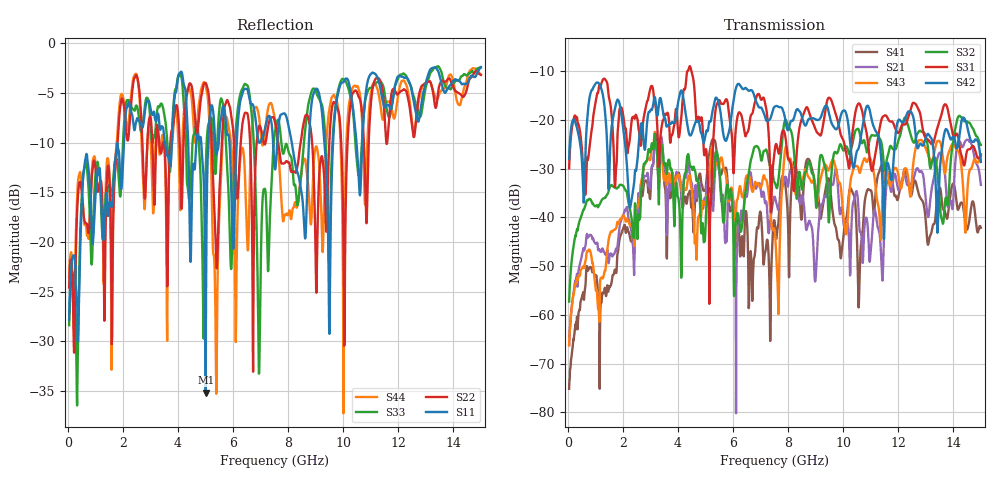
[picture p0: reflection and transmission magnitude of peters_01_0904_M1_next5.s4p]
# MHZ S RI R 50.00
! FREQ  S11  S12  S13  S14
!  S21  S22  S23  S24
!  S31  S32  S33  S34
!  S41  S42  S43  S44
!  REAL  IMAG  REAL  IMAG  REAL  IMAG  REAL  IMAG
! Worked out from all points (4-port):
!   1496 points, 50 MHz to 15 GHz, reference 50 ohm
!   strongest paths, dB at 50 MHz, 3.79 GHz, 7.53 GHz, 11.27 GHz, 15 GHz:
!     S42: -28.0, -20.4, -17.2, -23.2, -28.6
!     S31: -30.0, -23.1, -25.6, -23.5, -27.1
!     S32: -57.3, -31.0, -33.0, -23.4, -25.1
!     S43: -66.3, -31.2, -43.7, -37.5, -27.4
!     S21: -66.2, -32.4, -36.0, -42.3, -33.3
!     S41: -75.2, -32.0, -41.9, -31.2, -42.1
!   lowest |S11| = -35.2 dB at 5.01 GHz (marker M1), VSWR 1.04, Z = 49 + j1.41 ohm
!   |S11| at or under -10 dB: start of sweep to 2.042 GHz; 8.134 GHz to 8.756 GHz (622.5 MHz wide, 7.37 % of centre); 9.318 GHz to 9.633 GHz (314.2 MHz wide, 3.32 % of centre)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
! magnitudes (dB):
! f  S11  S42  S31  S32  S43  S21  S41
! 50 MHz  -27.9  -28.0  -30.0  -57.3  -66.3  -66.2  -75.2
! 3.15 GHz  -7.3  -15.3  -16.3  -23.3  -22.8  -24.0  -24.7
! 5.01 GHz  -35.2  -22.9  -26.1  -40.7  -37.2  -35.9  -34.1
! 5.38 GHz  -11.0  -15.4  -17.5  -26.6  -29.0  -28.4  -25.4
! 6.64 GHz  -6.1  -13.9  -19.3  -28.4  -33.0  -30.8  -46.9
! 8.72 GHz  -12.5  -20.1  -17.7  -28.8  -31.5  -41.5  -28.0
! 15 GHz  -2.4  -28.6  -27.1  -25.1  -27.4  -33.3  -42.1
